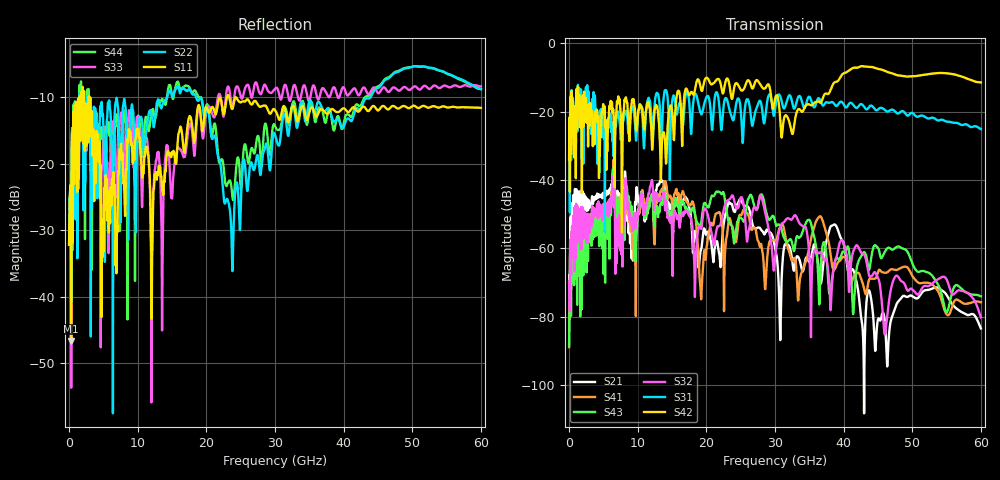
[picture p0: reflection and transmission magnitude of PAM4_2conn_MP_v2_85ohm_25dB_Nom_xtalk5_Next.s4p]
! Info: Touchstone file created by Circ.  Input file=FAB50GbE_2conn_Midplane_Examax_Topo2_v2_85ohm_25dB_Nom.circ
# Hz S RI R 50
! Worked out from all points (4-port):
!   6000 points, 10 MHz to 60 GHz, reference 50 ohm
!   strongest paths, dB at 10 MHz, 15.01 GHz, 30.01 GHz, 45.01 GHz, 60 GHz:
!     S42: -34.0, -19.7, -16.3, -7.5, -11.4
!     S31: -34.0, -17.1, -19.3, -19.4, -25.1
!     S32: -70.1, -55.2, -62.8, -68.6, -80.2
!     S43: -88.5, -53.4, -52.1, -59.9, -74.1
!     S41: -89.0, -47.5, -57.8, -67.0, -75.8
!     S21: -69.7, -50.7, -59.8, -80.9, -83.5
!   lowest |S11| = -46.7 dB at 310 MHz (marker M1), VSWR 1.01, Z = 50.3 + j0.316 ohm
!   |S11| at or under -10 dB: start of sweep to 1.521 GHz; 2.904 GHz to 23.01 GHz (20.11 GHz wide, 155 % of centre); 23.32 GHz to end of sweep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
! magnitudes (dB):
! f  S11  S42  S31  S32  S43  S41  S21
! 10 MHz  -32.2  -34.0  -34.0  -70.1  -88.5  -89.0  -69.7
! 310 MHz  -46.7  -21.5  -22.4  -66.3  -66.9  -67.1  -63.1
! 6.43 GHz  -21.7  -19.3  -30.7  -39.1  -37.2  -36.0  -38.8
! 19.22 GHz  -13.4  -13.4  -20.6  -54.1  -53.2  -74.4  -60.4
! 25.56 GHz  -10.7  -13.0  -20.3  -49.3  -51.8  -48.9  -47.7
! 30.72 GHz  -13.4  -21.0  -15.3  -54.2  -53.2  -53.9  -82.8
! 60 GHz  -11.6  -11.4  -25.1  -80.2  -74.1  -75.8  -83.5
